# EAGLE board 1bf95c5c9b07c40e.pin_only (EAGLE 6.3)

Size 19.05 x 19.05 mm. Coordinates in mm from the lower left corner, seen from the top.
Outline: 19.05,16.51 19.05,2.54 arc-90 16.51,0 2.54,0 arc-90 0,2.54 0,16.51 arc-90 2.54,19.05 16.51,19.05 arc-90 19.05,16.51
Copper layers (1*16): Top 0.035mm / dielectric 1.5mm / Bottom 0.035mm
Design rules "default": minimum track width 8mil, minimum drill 0.4mm, track to track 8mil, track to pad 8mil, pad to pad 8mil, via to via 8mil, smd to smd 8mil, copper to edge 20mil, drill to drill 8mil, minimum pad ring 8mil, minimum via ring 10mil, stop-mask expansion 3mil, vias tented up to drill 20mil, thermal gap 8mil
tRestrict: area 12.4,25.5 to 12.8,25.6; area 10.1,23.1 to 10.5,23.5; area 11.2,23.1 to 11.5,23.5; area 9.6,24 to 10,24.4

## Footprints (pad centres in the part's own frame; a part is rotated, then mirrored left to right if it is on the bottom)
_0805 = smd 1.2 x 1.3: 1 -1.016,0; 2 1.016,0
FIDUCIAL_1MM = smd 1 x 1: 1 0,0
1X07_ROUND_70 = drill 1 pad 1.778 square: 1 -7.62,0 | drill 1 pad 1.778: 2 -5.08,0; 3 -2.54,0; 4 0,0; 5 2.54,0; 6 5.08,0; 7 7.62,0
LFCSP16_LQ = smd 0.8 x 0.25: 1 -1.5,0.75; 2 -1.5,0.25; 3 -1.5,-0.25; 4 -1.5,-0.75; 9 1.5,-0.75; 10 1.5,-0.25; 11 1.5,0.25; 12 1.5,0.75 | smd 0.25 x 0.8: 5 -0.75,-1.5; 6 -0.25,-1.5; 7 0.25,-1.5; 8 0.75,-1.5; 13 0.75,1.5; 14 0.25,1.5; 15 -0.25,1.5; 16 -0.75,1.5
SOT23-5 = smd 0.55 x 1.2: 1 -0.95,-1.3; 2 0,-1.3; 3 0.95,-1.3; 4 0.95,1.3; 5 -0.95,1.3
MOUNTINGHOLE_2.5_PLATED = drill 2.5 pad 3.2: P$1 0,0

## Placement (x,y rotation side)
C1  0.01uF  [_0805]  5.84,11.81 90 top
C2  0.01uF  [_0805]  8.89,8.38 180 top
C3  0.01uF  [_0805]  13.46,11.68 90 top
C4  10µF  [_0805]  12.06,6.22 270 top
C5  10µF  [_0805]  5.71,6.86 270 top
FID1  FIDUCIAL""  [FIDUCIAL_1MM]  1.63,13.44 0 top
FID2  FIDUCIAL""  [FIDUCIAL_1MM]  17.78,9.4 0 top
FID3  FIDUCIAL""  [FIDUCIAL_1MM]  11.68,9.53 0 top
JP2  [1X07_ROUND_70]  9.53,1.91 0 top
U1  ADXL377  [LFCSP16_LQ]  9.53,12.07 90 top
U2  RT9193  [SOT23-5]  8.89,5.84 270 top
U$2  MOUNTINGHOLE2.5  [MOUNTINGHOLE_2.5_PLATED]  16.51,16.51 0 top
U$3  MOUNTINGHOLE2.5  [MOUNTINGHOLE_2.5_PLATED]  2.54,16.51 0 top
U$16  [ADAFRUIT_2.5MM]  0.89,9.14 0 top
U$17  MOUNTINGHOLE2.5  [MOUNTINGHOLE_2.5_PLATED]  2.54,6.35 0 top
U$18  MOUNTINGHOLE2.5  [MOUNTINGHOLE_2.5_PLATED]  16.51,6.35 0 top
U$19  [ADAFRUIT_2.5MM]  10.79,4.83 0 bottom

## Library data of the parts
C1-C5 FID1-FID3 JP2 U1 U2 U$2 U$3 U$16-U$19 = microbuilder

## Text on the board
tPlace: ADXL377 | 3-Axis 200g | Y | X | Z | VIN | 3V | Z | Y | GND | T | X
bPlace: ADXL377 3-Axis | +-200g Accelerometer | VIN: 3.3-5V | Analog Output: 3.3V | adafruit!

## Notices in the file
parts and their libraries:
microbuilder: This work is placed in the public domain, and may be freely used for commercial and non-commercial work with the following conditions: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
